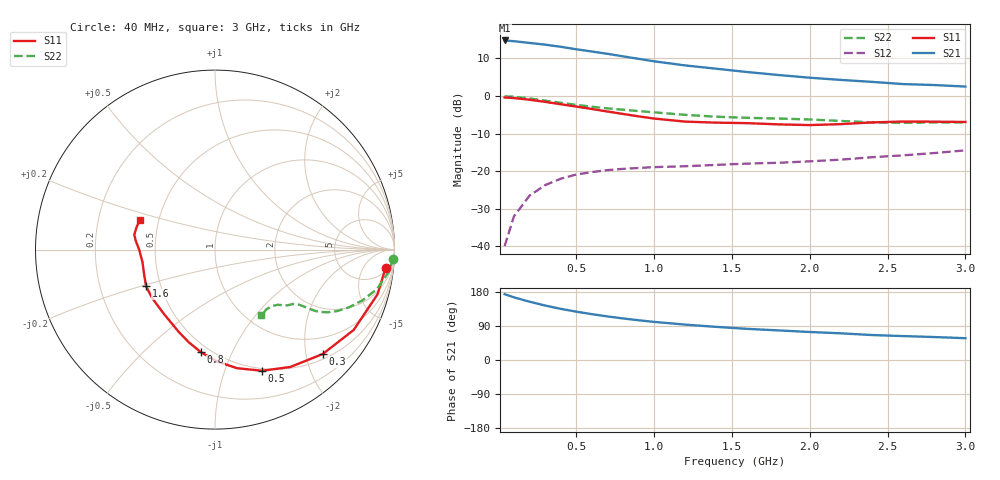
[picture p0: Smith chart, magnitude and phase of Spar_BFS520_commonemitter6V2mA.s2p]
! Filename:  BFS520G.S2P  Version:  4.0
! NXP part #: BFS520  Date: Jun 1994
! Bias condition: Vce=6V, Ic=2mA
#  MHz  S  MA  R  50
! Freq  S11  S21  S12  S22  !GUM [dB]
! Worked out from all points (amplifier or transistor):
!   21 points, 40 MHz to 3 GHz, reference 50 ohm
!   highest |S21| = 14.8 dB at 40 MHz (marker M1)
!   |S21| within 3 dB of that: start of sweep to 609.1 MHz
!   unconditionally stable (mu >= 1): 1.359 GHz to end of sweep
!   at 300 MHz: K = 0.28, MSG = 18.7 dB, |S12| = -23.7 dB
!   at 1 GHz: K = 0.77, MSG = 14.1 dB, |S12| = -18.9 dB
!   at 3 GHz: K = 1.21, MAG = 5.7 dB, |S12| = -14.5 dB
!   S11 on the Smith chart (normalised r, x): 40 MHz: 7, -16; 300 MHz: 0.60, -2.34; 500 MHz: 0.48, -1.35; 800 MHz: 0.45, -0.77; 1.6 GHz: 0.41, -0.21; 3 GHz: 0.39, +0.16
40  0.956 -6.2  5.495 173.7  0.01 86.1  0.992 -2.9
100  0.939 -15.4  5.368 165.4  0.025 79.2  0.977 -7.2
200  0.893 -30.1  5.096 153.8  0.047 70.1  0.929 -13.7
300  0.836 -44.1  4.834 143.8  0.065 62.8  0.869 -19.0
400  0.777 -57.3  4.527 135.0  0.079 57.3  0.813 -23.3
500  0.724 -68.8  4.196 127.6  0.09 52.8  0.762 -26.7
600  0.672 -79.5  3.915 121.0  0.097 49.9  0.72 -29.0
700  0.622 -89.3  3.65 115.0  0.103 47.9  0.685 -30.5
800  0.577 -97.8  3.375 109.7  0.107 46.6  0.657 -31.4
900  0.536 -105.9  3.13 104.9  0.11 45.7  0.63 -31.9
1000  0.501 -113.8  2.899 100.6  0.113 45.2  0.606 -32.3
1200  0.456 -129.4  2.555 93.4  0.116 45.5  0.561 -33.2
1400  0.442 -142.4  2.309 87.4  0.121 47.2  0.53 -34.9
1600  0.435 -151.9  2.085 82.1  0.126 49.4  0.512 -37.2
1800  0.419 -160.3  1.903 78.1  0.129 52.7  0.501 -38.5
2000  0.41 -170.2  1.753 73.9  0.135 56.0  0.487 -39.5
2200  0.422 -179.8  1.638 70.4  0.142 59.7  0.465 -41.4
2400  0.445 173.5  1.543 65.9  0.153 62.7  0.446 -44.9
2600  0.457 169.6  1.442 63.1  0.162 65.2  0.439 -49.5
2800  0.455 165.0  1.4 60.6  0.174 68.3  0.445 -52.9
3000  0.451 158.5  1.336 57.5  0.189 70.6  0.446 -54.7
